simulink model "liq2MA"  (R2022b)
settings: Solver=ode45  StartTime=0.0  StopTime=600*5  FixedStep=1  RelTol=1e-6  EnableMultiTasking=on
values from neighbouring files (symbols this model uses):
  a = k12/(2*Ar*sqrt(h1b-h2b))    [para2Kp.m]    (also in nyqlog.m = log(spiralfactor)*2/pi)
  Ar = 6*25.4    (= 152.4)    [para2Kp.m]
  b = k2/(2*Ar*sqrt(h2b))    [para2Kp.m]
  h2b = (qb/k2)^2    (= 5.00000710049)    [para2Kp.m]
  k1 = 0    [para2Kp.m]
  k12 = 38    [para2Kp.m]
  k2 = 11.5    [para2Kp.m]
  qb = 25.7148    [para2Kp.m]
  qmax = 90    [para2Kp.m]
  qmin = -85    [para2Kp.m]
libraries: simulink x1

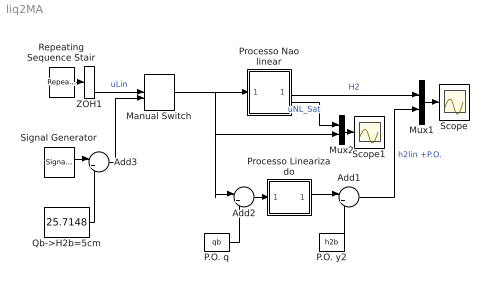
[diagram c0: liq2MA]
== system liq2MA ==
  Add1 : Sum  Inputs=|++
  Add2 : Sum  Inputs=|+-
  Add3 : Sum  Inputs=|++
  Manual Switch : ManualSwitch
  Mux1 : Mux  Inputs=2
  Mux2 : Mux  Inputs=2
  P.O. q : Constant  Value=qb
  P.O. y2 : Constant  Value=h2b
  Processo Linearizado : Subsystem
  Processo Nao linear : Subsystem
  Qb->H2b=5cm : Constant  Value=25.7148
  Repeating Sequence Stair : simulink/Sources/Repeating Sequence Stair  OutValues=25.7148*[2 5 20 5 2]/5.'  tsamp=500  OutMin=[]  OutMax=[]  OutDataTypeStr=double  OutputDataTypeScalingMode=double  OutDataType=fixdt(0,8)  ConRadixGroup=Best Precision: Vector-wise  OutScaling=2^-12
  Scope : Scope
  Scope1 : Scope
  Signal Generator : SignalGenerator  WaveForm=square  Amplitude=20  Frequency=1/1000
  ZOH1 : ZeroOrderHold
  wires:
  Mux1/1 -> Scope/1
  Repeating Sequence Stair/1 -> ZOH1/1
  Processo Linearizado/1(h2) -> Add1/1
  Mux2/1 -> Scope1/1
  Processo Nao linear/3("Usat ") -> Mux2/1  "uNL_Sat"
  Add1/1 -> Mux1/2  "h2lin +P.O."
  P.O. q/1 -> Add2/2
  Add2/1 -> Processo Linearizado/1(ul)
  P.O. y2/1 -> Add1/2
  Manual Switch/1 -> Add2/1, Mux2/2, Processo Nao linear/1(u)
  Qb->H2b=5cm/1 -> Add3/2
  Signal Generator/1 -> Add3/1
  ZOH1/1 -> Manual Switch/1  "uLin"
  Add3/1 -> Manual Switch/2
  Processo Nao linear/2(H2) -> Mux1/1  "H2"

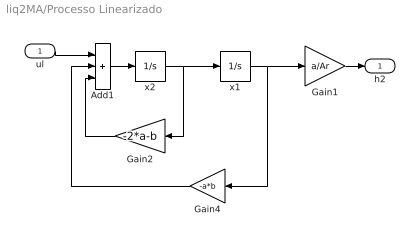
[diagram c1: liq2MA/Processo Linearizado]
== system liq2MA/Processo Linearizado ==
  ul : Inport
  Add1 : Sum  Inputs=+++
  Gain1 : Gain  Gain=a/Ar
  Gain2 : Gain  Gain=-2*a-b
  Gain4 : Gain  Gain=-a*b
  x1 : Integrator  InitialCondition=5
  x2 : Integrator  InitialCondition=6
  h2 : Outport
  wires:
  ul/1 -> Add1/1
  x1/1 -> Gain1/1, Gain4/1
  x2/1 -> Gain2/1, x1/1
  Gain1/1 -> h2/1
  Add1/1 -> x2/1
  Gain2/1 -> Add1/3
  Gain4/1 -> Add1/2

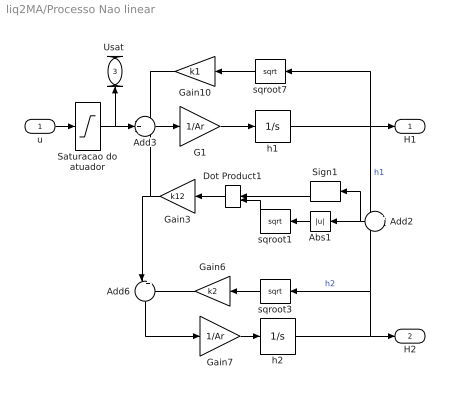
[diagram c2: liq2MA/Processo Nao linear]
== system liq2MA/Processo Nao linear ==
  u : Inport
  Abs1 : Abs
  Add2 : Sum  Inputs=+-
  Add3 : Sum  Inputs=-+-
  Add6 : Sum  Inputs=|+-
  Dot Product1 : DotProduct
  G1 : Gain  Gain=1/Ar
  Gain10 : Gain  Gain=k1
  Gain3 : Gain  Gain=k12
  Gain6 : Gain  Gain=k2
  Gain7 : Gain  Gain=1/Ar
  Saturacao do atuador : Saturate  UpperLimit=qmax  LowerLimit=qmin
  Sign1 : Signum
  h1 : Integrator  InitialCondition=5  LimitOutput=on  UpperSaturationLimit=16.5  LowerSaturationLimit=0
  h2 : Integrator  InitialCondition=6  LimitOutput=on  UpperSaturationLimit=16.5  LowerSaturationLimit=0
  sqroot1 : Math  Operator=sqrt  SignedPower=on
  sqroot3 : Math  Operator=sqrt  SignedPower=on
  sqroot7 : Math  Operator=sqrt  SignedPower=on
  H1 : Outport
  H2 : Outport  Port=2
  "Usat " : Outport  Port=3
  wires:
  h1/1 -> Add2/1, H1/1, sqroot7/1  "h1"
  h2/1 -> Add2/2, sqroot3/1, H2/1  "h2"
  Saturacao do atuador/1 -> "Usat "/1, Add3/2
  Add6/1 -> Gain7/1
  Gain10/1 -> Add3/1
  sqroot7/1 -> Gain10/1
  Gain6/1 -> Add6/2
  Gain7/1 -> h2/1
  sqroot3/1 -> Gain6/1
  G1/1 -> h1/1
  Gain3/1 -> Add6/1, Add3/3
  Add3/1 -> G1/1
  Dot Product1/1 -> Gain3/1
  sqroot1/1 -> Dot Product1/2
  Sign1/1 -> Dot Product1/1
  Abs1/1 -> sqroot1/1
  Add2/1 -> Abs1/1, Sign1/1
  u/1 -> Saturacao do atuador/1
